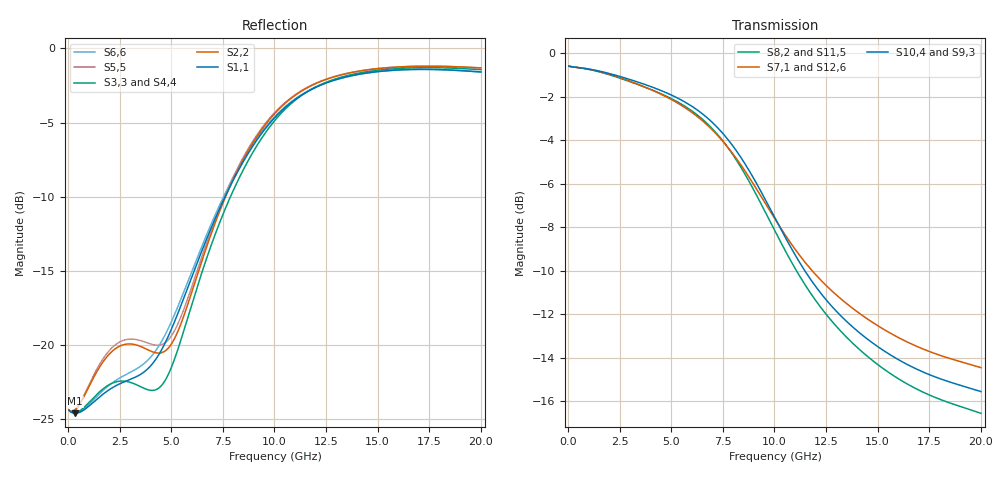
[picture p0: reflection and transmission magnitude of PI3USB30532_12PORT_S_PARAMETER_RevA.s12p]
! NPort=12 DATA=800 NOISE=0 GROUPDELAY=0 COMPLEX_DATAFORMAT=POLAR
! NumOfBlock=1 NumOfParam=0
! .MODEL Smodel S TSTONEFILE=PI3USB30532_12PORT_S_PARAMETER_RevA.s12p TYPE=S
!  -- The above .MODEL line can be used for the S element in the netlist.
! PORT DEFINITION
! PORT1 = TX+
! PORT2 = TX-
! PORT3 = RX+
! PORT4 = RX-
! PORT5 = DP0+
! PORT6 = DP0-
! PORT7 = TX1+
! PORT8 = TX1-
! PORT9 = RX1+
! PORT10 = RX1-
! PORT11 = RX2+
! PORT12 = RX2-
# Hz S MA R  50
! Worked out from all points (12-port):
!   800 points, 50 MHz to 20 GHz, reference 50 ohm
!   strongest paths, dB at 50 MHz, 5.044 GHz, 10.04 GHz, 15.03 GHz, 20 GHz:
!     S10,4: -0.6, -1.9, -7.6, -13.5, -15.5
!     S9,3: -0.6, -1.9, -7.6, -13.5, -15.5
!     S7,1: -0.6, -2.2, -7.6, -12.5, -14.5
!     S12,6: -0.6, -2.2, -7.7, -12.5, -14.4
!     S8,2: -0.6, -2.1, -8.2, -14.3, -16.5
!     S11,5: -0.6, -2.2, -8.3, -14.3, -16.5
!   lowest |S11| = -24.6 dB at 349.6 MHz (marker M1), VSWR 1.12, Z = 55.7 - j2.52 ohm
!   |S11| at or under -10 dB: start of sweep to 7.609 GHz
